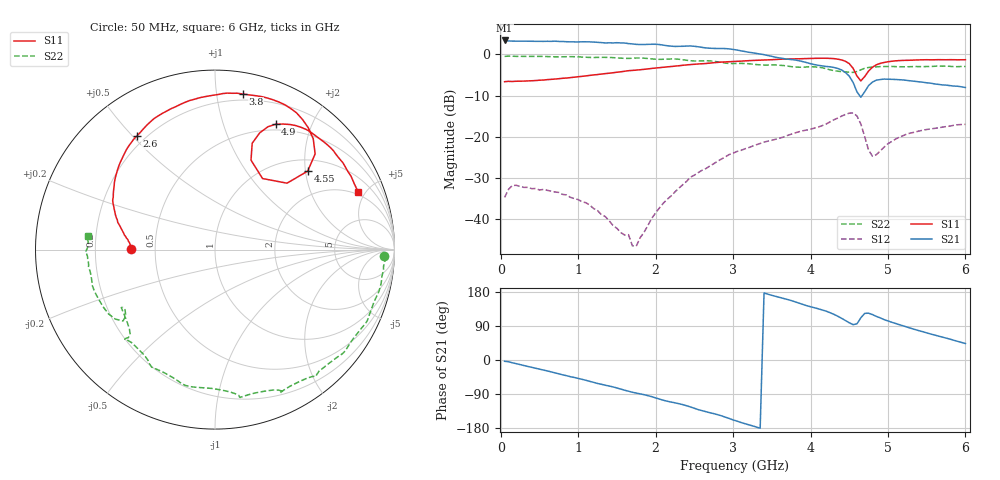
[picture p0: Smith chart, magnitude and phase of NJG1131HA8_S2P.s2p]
!S parameter
! Frequency  S11  S21  S12  S22
# HZ  S  DB R 50
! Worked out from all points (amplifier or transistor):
!   120 points, 50 MHz to 6 GHz, reference 50 ohm
!   highest |S21| = 3.4 dB at 50 MHz (marker M1)
!   |S21| within 3 dB of that: start of sweep to 3.255 GHz
!   unconditionally stable (mu >= 1): start of sweep to 2.914 GHz; 4.305 GHz to end of sweep
!   at 1.05 GHz: K = 2.61, MAG = 12.4 dB, |S12| = -35.8 dB
!   at 3.05 GHz: K = 0.90, MSG = 12.3 dB, |S12| = -23.6 dB
!   at 6 GHz: K = 1.78, MAG = -0.7 dB, |S12| = -17.0 dB
!   lowest NFmin = 0.40 dB at 10 MHz
!   S11 on the Smith chart (normalised r, x): 50 MHz: 0.36, +0.00; 2.6 GHz: 0.17, +0.51; 3.8 GHz: 0.15, +1.18; 4.55 GHz: 1.27, +2.06; 4.9 GHz: 0.43, +1.51; 6 GHz: 1.82, +4.46
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5e7  -6.64 179.7  3.36 -3.4  -34.70 -1.1  -0.50 -2.3
2e8  -6.53 177.5  3.19 -9.6  -31.76 -3.9  -0.50 -5.5
6e8  -6.14 173.0  3.16 -28.8  -32.97 -14.3  -0.55 -15.6
1.05e9  -5.34 166.7  3.04 -50.9  -35.75 -23.0  -0.67 -28.2
1.5e9  -4.35 158.0  2.82 -73.8  -42.19 -28.9  -0.87 -42.0
1.75e9  -3.83 151.7  2.41 -87.2  -46.52 134.7  -0.89 -51.5
2.05e9  -3.24 143.3  2.37 -103.1  -37.22 114.0  -1.23 -61.2
2.35e9  -2.67 133.2  1.95 -117.8  -31.63 107.1  -1.31 -65.6
2.6e9  -2.29 124.6  1.68 -133.7  -28.11 98.5  -1.59 -79.2
2.8e9  -1.96 116.7  1.42 -144.2  -25.93 92.2  -1.82 -82.0
3.05e9  -1.70 107.3  1.05 -161.3  -23.56 81.0  -2.22 -98.1
3.45e9  -1.35 92.5  -0.30 173.7  -21.05 64.4  -2.60 -115.7
3.8e9  -1.11 79.9  -1.36 153.6  -19.06 51.6  -3.07 -126.3
4.05e9  -0.98 71.0  -2.49 137.9  -17.90 40.6  -3.04 -135.1
4.4e9  -1.36 52.6  -3.78 110.2  -15.01 17.1  -4.20 -146.8
4.55e9  -3.39 40.3  -6.81 93.3  -14.22 -9.7  -4.39 -146.2
4.65e9  -6.44 56.2  -10.41 111.4  -16.90 -37.5  -3.76 -142.2
4.7e9  -5.40 68.1  -9.06 123.1  -19.97 -43.0  -3.39 -145.1
4.8e9  -3.13 69.0  -6.74 119.8  -24.71 -17.8  -3.10 -152.8
4.9e9  -2.20 64.2  -6.12 111.1  -23.43 5.8  -2.99 -159.7
5.05e9  -1.68 57.0  -6.07 99.5  -21.12 11.6  -2.95 -163.8
6e9  -1.32 21.9  -8.05 43.4  -16.97 -16.1  -2.96 173.8
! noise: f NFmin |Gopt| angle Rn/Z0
1e+07  0.3979  0.9754  0.2528  3.829
1.2e+08  0.5149  0.5882  6.614  0.2232
2.3e+08  0.553  0.5324  13.69  0.2006
3.4e+08  0.5975  0.4972  20.75  0.1943
4.5e+08  0.6522  0.4617  28  0.1899
5.6e+08  0.7154  0.4251  35.56  0.1855
6.7e+08  0.7854  0.3886  43.56  0.1808
7.8e+08  0.8606  0.3535  52.14  0.1757
8.9e+08  0.9398  0.321  61.43  0.1701
1e+09  1.022  0.2923  71.53  0.1643
